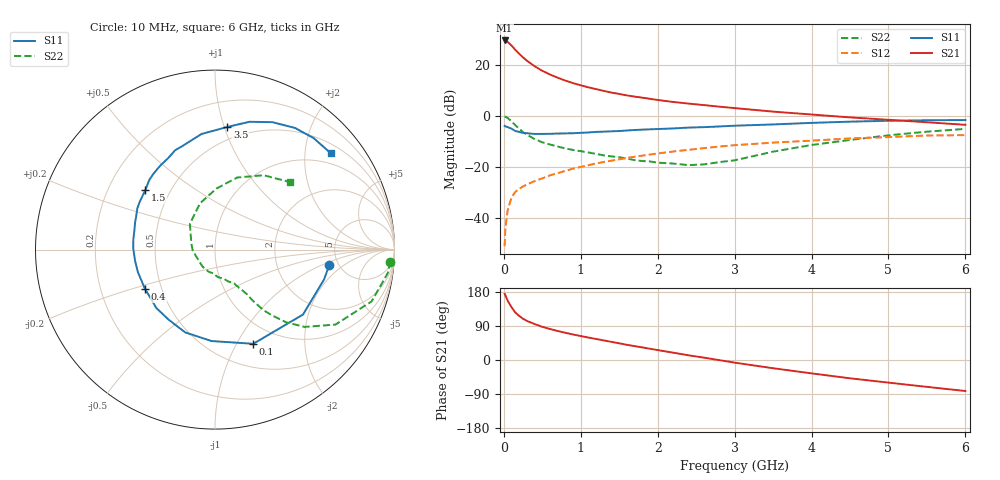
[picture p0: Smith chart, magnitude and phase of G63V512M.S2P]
! SIEMENS Small Signal Semiconductors
! BFG193
! Si NPN RF Bipolar Junction Transistor in SOT223
! VCE = 3.5 V  IC = 12 mA
! Common Emitter S-Parameters:  August  1996
# GHz  S  MA  R  50
!  f  S11  S21  S12  S22
! GHz  MAG  ANG  MAG  ANG  MAG  ANG  MAG  ANG
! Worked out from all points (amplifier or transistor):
!   36 points, 10 MHz to 6 GHz, reference 50 ohm
!   highest |S21| = 29.7 dB at 10 MHz (marker M1)
!   |S21| within 3 dB of that: start of sweep to 129.3 MHz
!   unconditionally stable (mu >= 1): 816.5 MHz to 2.515 GHz
!   at 250 MHz: K = 0.60, MSG = 25.3 dB, |S12| = -27.6 dB
!   at 1.4 GHz: K = 1.06, MAG = 11.8 dB, |S12| = -17.5 dB
!   at 6 GHz: K = 0.88, MSG = 2.0 dB, |S12| = -7.5 dB
!   S11 on the Smith chart (normalised r, x): 10 MHz: 4.21, -1.24; 100 MHz: 0.76, -1.17; 400 MHz: 0.40, -0.22; 1.5 GHz: 0.36, +0.32; 3.5 GHz: 0.40, +1.03; 6 GHz: 0.71, +2.59
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0.01  0.6426 -7.7  30.6 174.8  0.0028 86.3  0.9799 -3.9
0.02  0.63 -15.3  30.22 170.8  0.0062 84.0  0.9718 -7.7
0.05  0.6095 -36.4  28.59 156.3  0.0142 74.6  0.919 -18.3
0.1  0.5664 -67.9  24.34 139.3  0.0255 65.0  0.7906 -31.9
0.15  0.5099 -92.1  19.95 125.1  0.0326 56.7  0.6594 -40.8
0.2  0.4903 -109.8  16.76 116.2  0.0375 54.7  0.5649 -45.7
0.25  0.4681 -123.6  14.16 108.8  0.0416 52.4  0.4847 -49.1
0.3  0.4611 -135.1  12.24 103.2  0.0456 52.3  0.4331 -51.3
0.4  0.4472 -150.7  9.553 94.9  0.053 52.7  0.3544 -53.5
0.5  0.4477 -163.7  7.754 87.5  0.0601 53.0  0.3061 -54.4
0.6  0.4498 -172.1  6.567 81.9  0.0687 53.3  0.277 -55.9
0.7  0.4551 179.7  5.681 76.5  0.076 53.5  0.2531 -57.7
0.9  0.4614 166.9  4.455 67.3  0.093 52.7  0.2165 -60.5
1.1  0.4776 156.6  3.675 59.3  0.1089 51.3  0.1934 -67.1
1.5  0.51 139.6  2.727 44.1  0.1421 45.9  0.1559 -82.9
1.7  0.5342 133.2  2.419 36.6  0.1593 43.1  0.1367 -91.2
2.2  0.5729 117.0  1.898 19.4  0.2019 33.6  0.1173 -126.6
3  0.6486 96.6  1.438 -7.0  0.269 17.3  0.1357 165.9
3.5  0.6869 84.2  1.227 -21.7  0.3021 5.1  0.2009 134.2
4.5  0.7789 65.7  0.945 -48.3  0.3647 -14.7  0.3404 88.6
5.5  0.8294 48.5  0.758 -70.9  0.4164 -38.7  0.4952 56.8
6  0.8391 39.8  0.676 -81.8  0.4232 -52.6  0.5619 42.0
